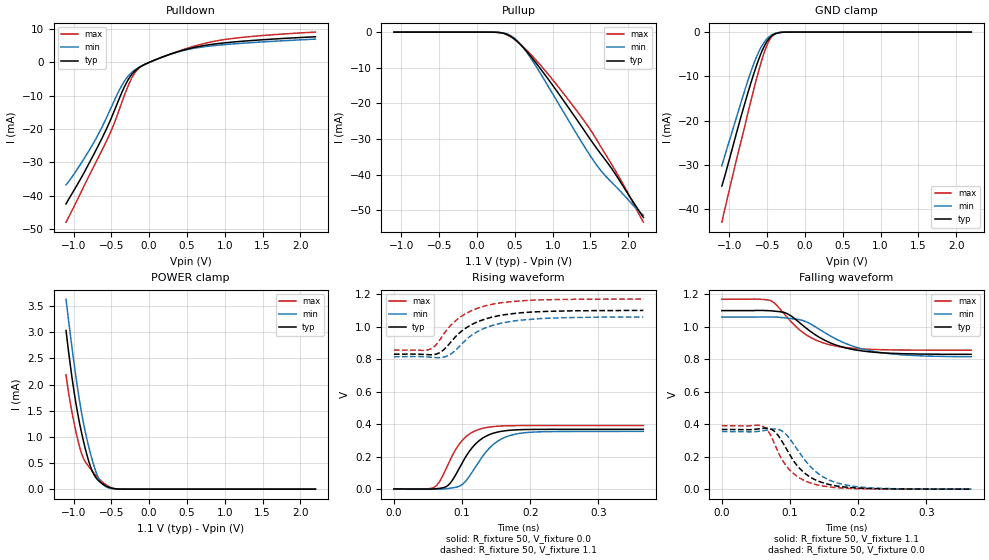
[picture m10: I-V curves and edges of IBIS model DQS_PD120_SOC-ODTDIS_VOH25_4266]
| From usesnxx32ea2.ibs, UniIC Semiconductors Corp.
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| DQS_PD120_SOC-ODTDIS_VOH25_4266
| (120 Ohm Pulldown, SOC ODT disabled setting, VOH=VDDQ/2.5 cal. point, 3200-4266Mbps)
[Model]   DQS_PD120_SOC-ODTDIS_VOH25_4266
Model_type   I/O
Vinl = 160.000mV
Vinh = 280.000mV
Vmeas = 220.000mV
Vref = 0.0mV
Cref = 0.0pF
|   typ   min   max
|C_comp   0.849pF   0.799pF   0.899pF
C_comp_pullup   0.4245pF   0.3995pF   0.4495pF
C_comp_pulldown   0.4245pF   0.3995pF   0.4495pF
| Note: C_comp changes when the ODT circuit is enabled.
[Model Spec]
| Input threshold voltage corners
Vinl   0.1600V   0.1520V   0.1740V
Vinh   0.2800V   0.2720V   0.2940V
| Measurement voltage corners
Vmeas   0.2200V   0.2120V   0.2340V
| Timing spec test load voltage corners
Vref   0.0000V   0.0000V   0.0000V
| Dynamic Overshoot Parameters from LPDDR4 Specification
D_overshoot_ampl_h   0.30   NA   NA
D_overshoot_ampl_l   0.30   NA   NA
D_overshoot_area_h   0.1n   NA   NA
D_overshoot_area_l   0.1n   NA   NA
[Voltage Range]   1.1000V   1.0600V   1.1700V
[Pullup Reference]   1.1000V   1.0600V   1.1700V
| Junction Temperature (Ambient temp is 35C typ 95C min -40C max)
[Temperature Range]   50.0   110.0   -40.0
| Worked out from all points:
|   slope of the pulldown table from 0 to 0.165 V, typ, clamps not added: 108 ohm
|   slope of the pullup table from 0 to 0.165 V, typ, clamps not added: 17.5 kohm
|   GND clamp passes 1 mA (typ) near -0.45 V on its own axis
|   POWER clamp passes 1 mA (typ) near -0.88 V on its own axis
|   rising waveform, R_fixture 50, V_fixture 0.0: 20-80 % time 35.3ps typ, 39.2ps min, 32.1ps max; typ from 0.001 V to 0.368 V
|   falling waveform, R_fixture 50, V_fixture 1.1: 20-80 % time 62ps typ, 72.3ps min, 51.9ps max; typ from 1.1 V to 0.831 V
|   rising waveform, R_fixture 50, V_fixture 1.1: 20-80 % time 53.9ps typ, 54.9ps min, 51.6ps max; typ from 0.83 V to 1.1 V
|   falling waveform, R_fixture 50, V_fixture 0.0: 20-80 % time 41.6ps typ, 46.3ps min, 36.8ps max; typ from 0.368 V to 0.001 V
[Pulldown]
|   Voltage   I(typ)   I(min)   I(max)
-1.1V     -42.5mA    -36.8mA    -48mA
-921.8mV  -35.59mA   -31.07mA   -39.98mA
-713.9mV  -26.83mA   -23.34mA   -30.43mA
-502.7mV  -16.83mA   -13.59mA   -20.58mA
-334.4mV  -7.726mA   -5.944mA   -10.35mA
-222.2mV  -3.417mA   -2.876mA   -4.404mA
-123.2mV  -1.45mA    -1.361mA   -1.547mA
0V        -29.6uA    -24.6uA    -21.53uA
378.4mV   3.16mA     3.086mA    3.283mA
837.1mV   5.412mA    4.961mA    6.196mA
1.269V    6.388mA    5.775mA    7.572mA
2.2V      7.669mA    6.972mA    9.07mA
[GND Clamp]
|   Voltage   I(typ)   I(min)   I(max)
-1.1V     -34.75mA   -30.2mA    -42.92mA
-1.047V   -31.66mA   -27.14mA   -39.03mA
-941.6mV  -25.02mA   -21.25mA   -31.33mA
-796.4mV  -16.12mA   -13.14mA   -21.2mA
-671mV    -9.083mA   -6.865mA   -12.51mA
-595.1mV  -5.401mA   -3.898mA   -7.694mA
-525.8mV  -2.769mA   -1.975mA   -3.966mA
-473mV    -1.423mA   -1.031mA   -1.887mA
-416.9mV  -599.5uA   -440.4uA   -665.5uA
-360.8mV  -205.9uA   -154.4uA   -188.6uA
-265.1mV  -19.58uA   -16.73uA   -12.32uA
2.2V      0A         0A         0A
[Pullup]
|   Voltage   I(typ)   I(min)   I(max)
-1.1V     4.106uA    7.431uA    1.361uA
262.9mV   -64.81uA   -63.79uA   -66.42uA
394.9mV   -632.2uA   -524.2uA   -750.4uA
507.1mV   -2.159mA   -1.948mA   -2.249mA
612.7mV   -4.374mA   -4.387mA   -4.193mA
748mV     -7.805mA   -8.519mA   -7.126mA
1.078V    -17.24mA   -20.1mA    -15.44mA
1.471V    -29.26mA   -33.86mA   -26.53mA
1.675V    -35.26mA   -39.82mA   -33.5mA
1.788V    -38.54mA   -42.33mA   -37.4mA
1.943V    -43.63mA   -45.77mA   -43.12mA
2.2V      -52.05mA   -51.41mA   -53.39mA
[POWER Clamp]
|   Voltage   I(typ)   I(min)   I(max)
-1.1V     3.033mA    3.633mA    2.184mA
-1.044V   2.381mA    2.967mA    1.653mA
-984.5mV  1.782mA    2.31mA     1.205mA
-908.6mV  1.177mA    1.582mA    748.2uA
-852.5mV  818.2uA    1.149mA    543.6uA
-776.6mV  434.2uA    683.3uA    390.2uA
-707.3mV  225.6uA    345.4uA    267.6uA
-654.5mV  142.7uA    170.4uA    185.9uA
-591.8mV  77.93uA    64.81uA    105.5uA
-489.5mV  17.77uA    10.84uA    22.44uA
-377.3mV  1.505uA    1.061uA    1.223uA
2.2V      0A         0A         0A
[Ramp]
|   typ   min   max
| 20% - 80%
dV/dt_r   220.43m/35.33p   212.79m/39.18p   234.55m/32.12p
dV/dt_f   161.60m/61.86p   146.48m/72.39p   188.40m/51.96p
| 25% - 75%
|dV/dt_r   183.69m/28.11p   177.32m/31.19p   195.46m/25.51p
|dV/dt_f   134.67m/49.10p   122.07m/57.51p   157.00m/41.27p
R_load = 50
[Rising Waveform]
R_fixture = 50
V_fixture = 0.0
|   Time   V(typ)   V(min)   V(max)
0s        972.3uV    804.8uV    709.7uV
58ps      1.078mV    20.99uV    9.264mV
67ps      4.781mV    -49.41uV   47.09mV
77ps      16.25mV    2.537mV    130.4mV
101ps     168mV      31.04mV    303.3mV
114ps     251.1mV    99.41mV    347.6mV
130ps     313.3mV    201.5mV    374.2mV
154ps     353mV      299.8mV    387.8mV
184ps     365.8mV    342.9mV    391.1mV
366ps     368.4mV    355.4mV    391.6mV
[Falling Waveform]
R_fixture   = 50
V_fixture   = 1.1
V_fixture_min = 1.06
V_fixture_max = 1.17
|   Time   V(typ)   V(min)   V(max)
0s        1.1V       1.06V      1.17V
71ps      1.099V     1.061V     1.162V
80ps      1.095V     1.06V      1.135V
94ps      1.085V     1.054V     1.067V
121ps     1.001V     1.036V     959.1mV
142ps     938.2mV    987.8mV    911.5mV
165ps     891.7mV    930.5mV    883.5mV
201ps     854.5mV    869.6mV    865.1mV
239ps     839mV      838mV      858.7mV
366ps     830.7mV    815.9mV    856mV
[Rising Waveform]
R_fixture   = 50
V_fixture   = 1.1
V_fixture_min = 1.06
V_fixture_max = 1.17
|   Time   V(typ)   V(min)   V(max)
0s        830.4mV    814.6mV    855.9mV
52ps      826.8mV    812.6mV    859.7mV
62ps      831.3mV    809.5mV    889mV
75ps      865.6mV    814.7mV    965.9mV
90ps      936.7mV    853.6mV    1.035V
106ps     992.8mV    920.1mV    1.082V
123ps     1.03V      970.6mV    1.114V
144ps     1.059V     1.007V     1.138V
214ps     1.092V     1.05V      1.165V
366ps     1.1V       1.06V      1.17V
[Falling Waveform]
R_fixture = 50
V_fixture = 0.0
|   Time   V(typ)   V(min)   V(max)
0s        368.5mV    355.6mV    391.7mV
57ps      373.8mV    358.4mV    392.5mV
74ps      366.4mV    370.4mV    312.3mV
87ps      304.2mV    362.1mV    192.3mV
100ps     209.8mV    309.3mV    117.2mV
117ps     116.4mV    207mV      62.57mV
138ps     56.5mV     108mV      29.17mV
164ps     23.64mV    46.46mV    11.7mV
201ps     7.431mV    14.69mV    3.582mV
366ps     1.046mV    960uV      738.7uV
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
